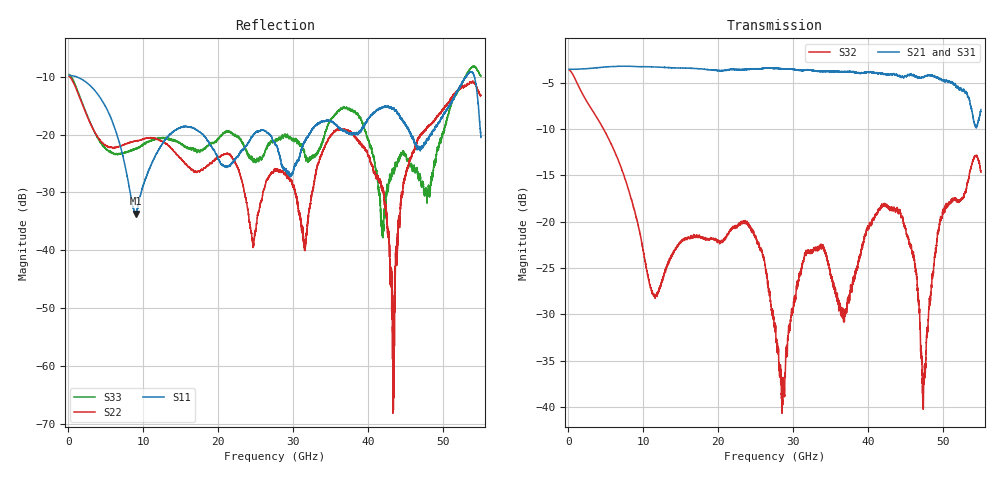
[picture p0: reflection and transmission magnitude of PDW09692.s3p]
!The following data was pulled from an Agilent PNA
!This sNp file was generated from the data in the RF Test software
!NOTE:  Smoothing/Math/Corrections applied on any given trace ARE included in the data saved here
# MHz S dB R 50
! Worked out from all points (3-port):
!   12801 points, 100 MHz to 55 GHz, reference 50 ohm
!   strongest paths, dB at 100 MHz, 13.82 GHz, 27.55 GHz, 41.27 GHz, 55 GHz:
!     S21: -3.6, -3.4, -3.5, -4.0, -7.9
!     S31: -3.6, -3.4, -3.5, -4.1, -7.4
!     S32: -3.6, -23.7, -31.6, -18.9, -14.7
!   lowest |S11| = -33.7 dB at 8.987 GHz (marker M1), VSWR 1.04, Z = 52 + j0.807 ohm
!   |S11| at or under -10 dB: 1.063 GHz to 52.99 GHz (51.93 GHz wide, 192 % of centre); 52.99355 GHz to 53.01303 GHz (19.48 MHz wide, 0.0367 % of centre); 54.13 GHz to end of sweep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
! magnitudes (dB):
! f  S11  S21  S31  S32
! 100 MHz  -9.8  -3.6  -3.6  -3.6
! 8.987 GHz  -33.7  -3.3  -3.3  -19.4
! 24.62 GHz  -20.1  -3.6  -3.6  -21.0
! 27.55 GHz  -21.5  -3.5  -3.5  -31.6
! 31.56 GHz  -21.2  -3.7  -3.7  -23.4
! 38.1 GHz  -19.8  -3.9  -4.1  -26.2
! 41.83 GHz  -15.3  -4.0  -4.1  -18.4
! 43.27 GHz  -15.4  -4.1  -4.2  -18.8
! 47.38 GHz  -21.7  -4.4  -4.1  -36.8
! 55 GHz  -20.5  -7.9  -7.4  -14.7
